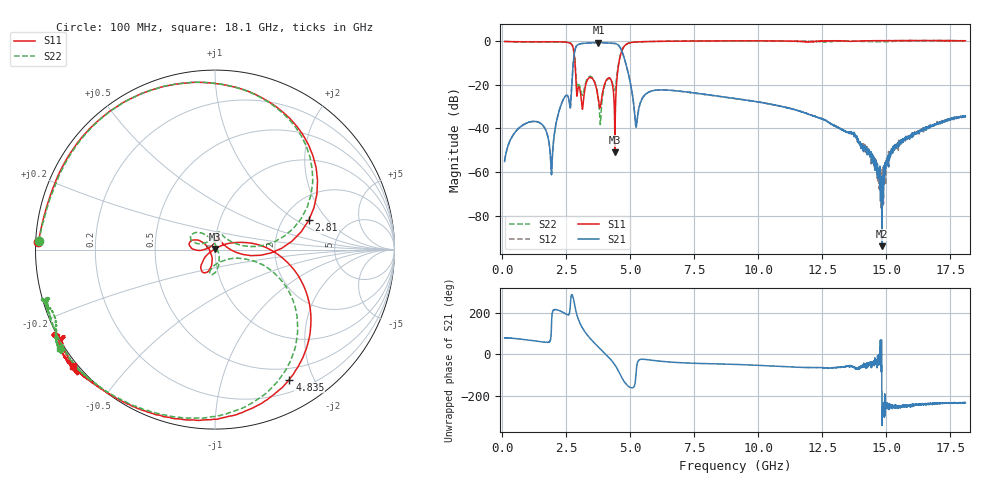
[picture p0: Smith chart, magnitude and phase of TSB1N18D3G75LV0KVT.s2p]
! TSB1N18D3G75LV0KVT  S-PARAMETER MODEL  ( General Type )
! Model Generated by TAIYO YUDEN Corporation (https://www.yuden.co.jp/en/)
! Version 1.0
! TAIYO YUDEN Control No. 20240527
! Copyright(c) 2024 TAIYO YUDEN CO.,LTD. All Rights Reserved.
! Products Name : Ceramic RF Devices
! Characteristics :
!  Passband freq : 3300-4200MHz ( At Passband , Insertion Loss : 1.5dB , VSWR 2.0 )
!  Attenuation : 15 dB min at 2500to 2690MHz, 10 dB min at 5150to 5925MHz, Impedance : 50 Ohm
!  Case Size : 1.6 x 0.8 / 0.063 x 0.031 [mm/inch] , Thickness : 0.65/ 0.026 [mm/inch]
!  (Conditions: Temperature = 25 degC , DC Bias Current/Voltage = 0A / 0V)
! External Node Assignments :
!  1  o---|-------|---o  2
!  |  BPF  |
! GND o---|-------|---o GND
! Frequency Range : 100MHz  -  18.1GHz  [ 3601 STEP ]
# MHZ S RI R 50
! Freq[MHz].  S11 Real  S11 Imag  S21 Real  S21 Imag  S12 Real  S12 Imag  S22 Real  S22 Imag
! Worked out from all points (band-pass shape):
!   3601 points, 100 MHz to 18.1 GHz, reference 50 ohm
!   highest |S21| = -0.65 dB at 3.765 GHz (marker M1); lowest = -94.1 dB at 14.84 GHz (marker M2)
!   |S21| within 3 dB of the highest: 2.857 GHz to 4.645 GHz (1.788 GHz wide, 47.7 % of centre)
!   lowest |S11| = -51.0 dB at 4.41 GHz (marker M3), VSWR 1.01, Z = 50 + j0.283 ohm
!   |S11| at or under -10 dB: 2.849 GHz to 4.564 GHz (1.714 GHz wide, 46.2 % of centre)
!   |S22| runs from -38.3 to 0.3 dB; largest |S21 - S12| = 0.0021
!   S11 on the Smith chart (normalised r, x): 100 MHz: 0.01, +0.02; 2.81 GHz: 2.75, +1.28; 4.835 GHz: 0.35, -1.67; 18.1 GHz: -0.01, -0.36
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100  -0.9839 0.0414  0.000287 0.00172  0.000362 0.00176  -0.9824 0.0452
1215  -0.8958 0.3615  0.00574 0.0133  0.00571 0.0132  -0.8815 0.3814
1935  -0.7421 0.6248  -0.000796 0.000348  -0.000803 0.000343  -0.726 0.6379
2245  -0.5632 0.7859  -0.0231 -0.0141  -0.023 -0.014  -0.553 0.791
2590  -0.0279 0.9286  -0.0505 -0.00944  -0.0507 -0.00949  -0.0492 0.9311
2810  0.5225 0.1635  -0.1024 -0.4382  -0.1025 -0.4374  0.5138 0.2367
2955  0.0185 0.0731  -0.8221 0.0172  -0.8227 0.0172  0.0361 0.086
3100  0.00166 0.0429  -0.6445 0.6005  -0.6444 0.5998  -0.0104 0.0627
3495  -0.1372 0.0455  0.312 0.8582  0.3109 0.8581  -0.1225 0.0887
3765  -0.0434 0.0158  0.7543 0.5406  0.754 0.5411  -0.01 0.0437
4165  -0.0638 -0.1287  0.8813 -0.2163  0.8804 -0.216  -0.0155 -0.139
4410  -0.000165 0.00283  0.5605 -0.6868  0.56 -0.6856  0.0437 -0.0633
4605  0.4136 -0.0817  -0.0479 -0.725  -0.0473 -0.7252  0.3884 -0.1968
4835  0.4148 -0.7238  -0.2388 -0.1909  -0.2389 -0.1914  0.3116 -0.7751
5240  -0.1254 -0.9487  0.0012 -0.0108  0.00119 -0.0107  -0.2048 -0.935
6100  -0.5131 -0.8472  0.0648 -0.0397  0.0649 -0.0398  -0.5565 -0.8192
9100  -0.7509 -0.6859  0.0322 -0.0357  0.0322 -0.0358  -0.7927 -0.6287
12100  -0.8378 -0.4872  0.00915 -0.0177  0.00927 -0.0178  -0.9419 -0.303
13770  -0.8663 -0.4999  0.0035 -0.00615  0.00289 -0.00648  -0.9529 -0.2832
14835  -0.8502 -0.579  -7.68e-07 -1.98e-05  0.000315 0.000493  -0.8917 -0.3748
15100  -0.8424 -0.6007  -0.000563 0.00242  -0.00135 0.00264  -0.8892 -0.421
18100  -0.7898 -0.6496  -0.0112 0.0152  -0.0114 0.0151  -0.8637 -0.5507
